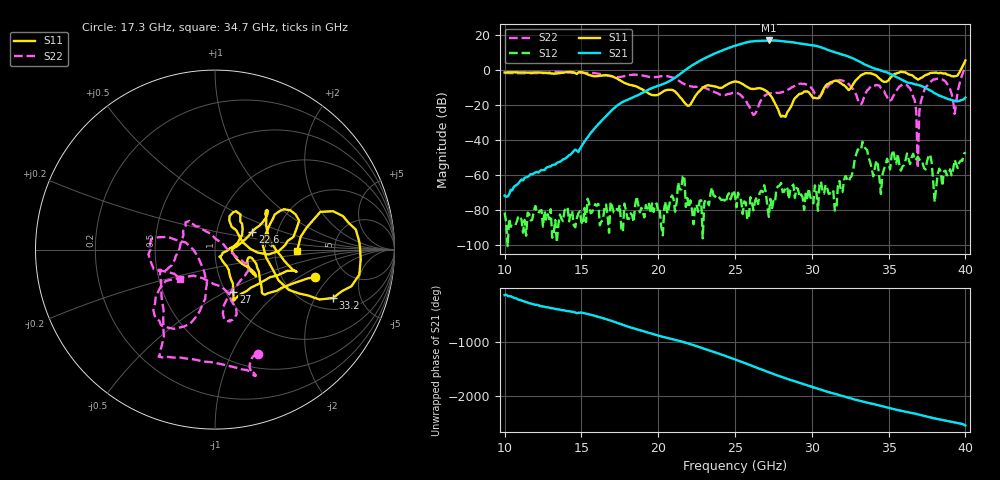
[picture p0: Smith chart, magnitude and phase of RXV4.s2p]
!Keysight Technologies,M9808A,MY58100618,A.14.70.03
!Date: Monday, February 27, 2023 13:44:28
!Correction: S11(Cdelta 2-Port  )
!S21(Cdelta 2-Port  )
!S12(Cdelta 2-Port  )
!S22(Cdelta 2-Port  )
!S2P File: Measurements: S11, S21, S12, S22:
# Hz S  RI  R 50
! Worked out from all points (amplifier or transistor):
!   301 points, 10 GHz to 40 GHz, reference 50 ohm
!   highest |S21| = 16.9 dB at 27.2 GHz (marker M1)
!   |S21| within 3 dB of that: 25.02 GHz to 30.2 GHz (5.188 GHz wide, 18.8 % of centre)
!   unconditionally stable (mu >= 1): start of sweep to 39.64 GHz
!   at 15 GHz: K = 126547.18, MAG = -32.4 dB, |S12| = -87.1 dB
!   at 25 GHz: K = 290.79, MAG = 15.2 dB, |S12| = -71.8 dB
!   at 40 GHz: K = 972.14, MSG = 15.7 dB, |S12| = -47.0 dB
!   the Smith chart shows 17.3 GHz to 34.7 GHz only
!   S11 on the Smith chart (normalised r, x): 17.3 GHz: 3.02, -1.40; 22.6 GHz: 1.48, +0.31; 27 GHz: 1.08, -0.55; 33.2 GHz: 2.60, -2.84; 34.7 GHz: 2.69, -0.04
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1e10  0.1542 0.8367  -0.000228 -0.000112  -6.33e-05 -5.39e-05  0.7101 0.4309
1.5e10  0.6894 0.5359  -0.00262 -0.00598  3.02e-05 -3.25e-05  0.6324 -0.5397
1.73e10  0.5564 -0.155  0.042 0.0842  7.85e-05 7.1e-05  0.2398 -0.5796
2e10  0.1808 -0.0769  -0.3517 -0.0516  -4.2e-05 7.12e-05  -0.2316 -0.6017
2.26e10  0.2078 0.1004  1.678 -0.4134  -5.12e-05 -7.15e-05  -0.3119 -0.1122
2.38e10  0.2861 0.1655  -1.839 -2.541  -0.000183 -0.000192  -0.2197 -0.0374
2.5e10  0.4552 -0.1235  -2.135 4.464  -0.000152 -0.000207  -0.1603 0.1543
2.56e10  0.3434 -0.1457  3.569 4.827  0.000174 7.63e-06  -0.085 0.128
2.61e10  0.1735 -0.2326  6.569 -0.2098  0.000114 -0.000114  0.00155 0.0615
2.7e10  0.1022 -0.2364  -1.031 -6.895  5.04e-05 -0.000317  0.1779 -0.077
2.72e10  0.1001 -0.1913  -3.444 -6.128  4.12e-05 4.73e-05  0.1853 -0.0977
2.78e10  0.0419 -0.0636  -6.89 0.1831  0.000444 0.000139  0.1518 -0.1611
2.86e10  0.0829 0.00757  -1.282 6.2  0.000165 -0.000337  0.0586 -0.2918
2.93e10  0.1412 0.1554  4.513 3.566  0.000276 -2.59e-05  0.0855 -0.3995
3e10  0.0798 0.1615  4.698 -2.15  -0.000164 -9e-05  0.0914 -0.2857
3.06e10  0.198 0.00339  0.7773 -4.419  0.000187 0.00062  -0.1213 -0.1449
3.14e10  0.4569 0.1242  -2.755 -1.903  4.37e-05 0.000338  -0.3344 -0.3018
3.32e10  0.6573 -0.2696  0.4701 1.592  4.41e-05 0.00528  -0.096 -0.0379
3.47e10  0.4582 -0.00533  0.8166 -0.39  -0.000897 0.00117  -0.1961 -0.1622
3.5e10  0.4678 -0.2139  0.5505 -0.5938  0.000314 -0.00201  -0.00216 -0.129
3.69e10  0.5119 -0.1416  -0.3657 -0.0886  -0.000296 0.00331  -0.00155 0.000246
4e10  1.132 -1.504  0.1614 -0.026  -0.0007 -0.00439  0.5762 -1.107
